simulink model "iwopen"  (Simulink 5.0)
settings: Solver=ode45  StartTime=0  StopTime=20  MaxStep=1e-3  RelTol=1e-3
undefined symbols (not defined in the file or in its folder): sat

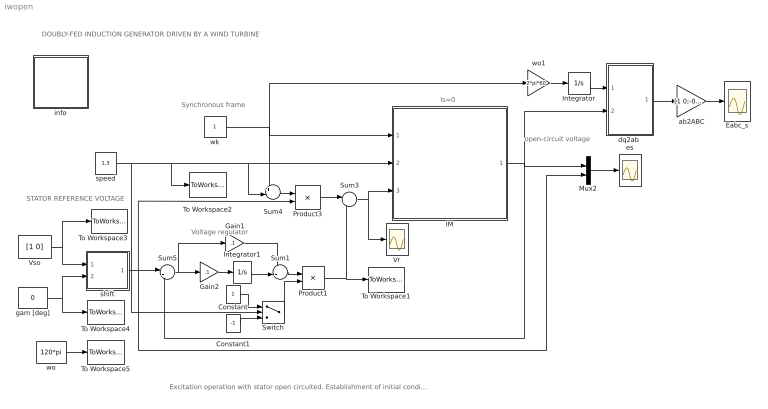
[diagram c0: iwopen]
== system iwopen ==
  note: STATOR REFERENCE VOLTAGE
  note: Synchronous frame
  note: DOUBLY-FED INDUCTION GENERATOR DRIVEN BY A WIND TURBINE
  note: Excitation operation with stator open circuited. Establishment of initial conditions.
  note: Is=0
  note: open-circuit voltage
  note: Voltage regulator
  Constant : Constant
  Constant1 : Constant  Value=-1
  Eabc_s : Scope
  Gain1 : Gain  Gain=.1
  Gain2 : Gain  Gain=.1
  IM : Subsystem  mask{Rr=.02, Lm=5, Lrl=0.1, wo=2*pi*60}
      mask prompts: Rr "Rotor resistance [pu]"; Lm "Magnetizing inductance [pu]"; Lrl "Rotor leakage inductance [pu]"; wo "base frequency [rad/s]"
  Integrator : Integrator
  Integrator1 : Integrator  UpperSaturationLimit=sat  LowerSaturationLimit=-sat
  Mux2 : Mux  Inputs=2
  Product1 : Product
  Product3 : Product
  Sum1 : Sum  Inputs=++|
  Sum3 : Sum  Inputs=|+-
  Sum4 : Sum  Inputs=+-|
  Sum5 : Sum  Inputs=|+-
  Switch : Switch  Criteria=u2 > Threshold  Threshold=1
  To Workspace1 : ToWorkspace  VariableName=vro  SampleTime=-1  SaveFormat=Array
  To Workspace2 : ToWorkspace  VariableName=wmo  SampleTime=-1  SaveFormat=Array
  To Workspace3 : ToWorkspace  VariableName=vso  SampleTime=-1  SaveFormat=Array
  To Workspace4 : ToWorkspace  VariableName=gamo  SampleTime=-1  SaveFormat=Array
  To Workspace5 : ToWorkspace  VariableName=wo  SampleTime=-1  SaveFormat=Array
  Vr : Scope
  Vso : Constant  Value=[1 0]
  ab2ABC : Gain  Gain=[1 0;-0.5 sqrt(3)/2;-0.5 -sqrt(3)/2]  Multiplication=Matrix(K*u)
  "dq2ab " : Subsystem
  es : Scope
  gam [deg] : Constant  Value=0
  info : Subsystem
  shift : Subsystem
  speed : Constant  Value=1.3
  wk : Constant
  wo : Constant  Value=120*pi
  wo1 : Gain  Gain=2*pi*60
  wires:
  IM/1(es) -> Sum5/2, Mux2/1, "dq2ab "/2(dq)
  Sum5/1 -> Gain2/1, Gain1/1
  speed/1 -> To Workspace2/1, IM/2(wm), Sum4/2, Switch/2
  wk/1 -> IM/1(wk), wo1/1, Sum4/1
  Vso/1 -> shift/1(vso), To Workspace3/1
  gam [deg]/1 -> shift/2(gama), To Workspace4/1
  wo/1 -> To Workspace5/1
  Gain2/1 -> Integrator1/1
  shift/1(vs) -> Mux2/2, Sum5/1, Product3/2
  Mux2/1 -> es/1
  Integrator1/1 -> Sum1/2
  Gain1/1 -> Sum1/1
  Constant/1 -> Switch/1
  Constant1/1 -> Switch/3
  Sum1/1 -> Product1/1
  Switch/1 -> Product1/2
  "dq2ab "/1(ab) -> ab2ABC/1
  ab2ABC/1 -> Eabc_s/1
  wo1/1 -> Integrator/1
  Integrator/1 -> "dq2ab "/1(thetas)
  Sum4/1 -> Product3/1
  Product3/1 -> Sum3/1
  Product1/1 -> Sum3/2, To Workspace1/1
  Sum3/1 -> IM/3(vr), Vr/1

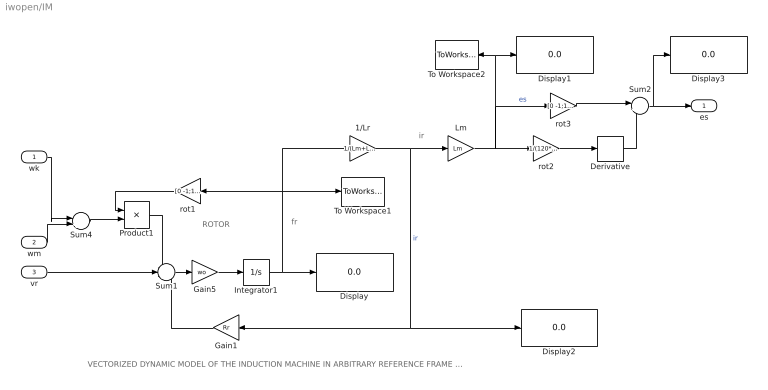
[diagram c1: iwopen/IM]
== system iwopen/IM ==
  note: ROTOR
  note: fr
  note: VECTORIZED DYNAMIC MODEL OF THE INDUCTION MACHINE IN ARBITRARY REFERENCE FRAME (stator open circuited --is=0)
  note: ir
  wk : Inport
  wm : Inport  Port=2
  vr : Inport  Port=3
  1/Lr : Gain  Gain=1/(Lm+Lrl)
  Derivative : Derivative
  Display{,1..3} (4 alike) : Display
  Gain1 : Gain  Orientation=left  Gain=Rr
  Gain5 : Gain  Gain=wo
  Integrator1 : Integrator  InitialCondition=[0 -1]
  Lm : Gain  Gain=Lm
  Product1 : Product
  Sum1 : Sum  Inputs=-+-
  Sum2 : Sum  Inputs=|++
  Sum4 : Sum  Inputs=|+-
  To Workspace1 : ToWorkspace  VariableName=fro  SampleTime=-1  SaveFormat=Array
  To Workspace2 : ToWorkspace  VariableName=fso  SampleTime=-1  SaveFormat=Array
  rot1 : Gain  Orientation=left  Gain=[0 -1;1 0]  Multiplication=Matrix(K*u)
  rot2 : Gain  Gain=1/(120*pi)  Multiplication=Matrix(K*u)
  rot3 : Gain  Gain=[0 -1;1 0]  Multiplication=Matrix(K*u)
  es : Outport
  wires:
  Gain1/1 -> Sum1/3
  Integrator1/1 -> rot1/1, To Workspace1/1, 1/Lr/1, Display/1
  Product1/1 -> Sum1/1
  rot1/1 -> Product1/1
  Sum4/1 -> Product1/2
  Sum1/1 -> Gain5/1
  Gain5/1 -> Integrator1/1
  wk/1 -> Sum4/1
  wm/1 -> Sum4/2
  vr/1 -> Sum1/2
  Lm/1 -> Display1/1, To Workspace2/1, rot3/1, rot2/1  "es"
  Sum2/1 -> es/1, Display3/1
  rot3/1 -> Sum2/1
  Derivative/1 -> Sum2/2
  rot2/1 -> Derivative/1
  1/Lr/1 -> Lm/1, Gain1/1, Display2/1  "ir"

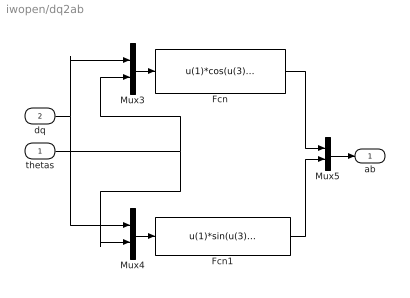
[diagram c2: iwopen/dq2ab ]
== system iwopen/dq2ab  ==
  thetas : Inport
  dq : Inport  Port=2
  Fcn : Fcn  Expr=u(1)*cos(u(3))-u(2)*sin(u(3))
  Fcn1 : Fcn  Expr=u(1)*sin(u(3))+u(2)*cos(u(3))
  Mux3 : Mux  Inputs=2
  Mux4 : Mux  Inputs=2
  Mux5 : Mux  Inputs=2
  ab : Outport
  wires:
  Mux3/1 -> Fcn/1
  Mux4/1 -> Fcn1/1
  dq/1 -> Mux3/1, Mux4/1
  thetas/1 -> Mux3/2, Mux4/2
  Fcn1/1 -> Mux5/2
  Fcn/1 -> Mux5/1
  Mux5/1 -> ab/1

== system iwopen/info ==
  note: The induction machine runs at a specified speed with the stator disconnected from the grid (is=0). The rotor is suddenly excited with slip-frequency voltages derived from voltage regulators so as to produce a commanded open-circuit stator terminal voltage. The induction machine is modeled in vectorized form in the synchronous frame . The specified operating conditions and the final values of the variables reached in a dc steady state are all saved in the workspace to serve as initial conditions in a subsequent simulation. This simulation deals with the connection of the stator to the grid.
  note: Doubly-Fed Induction Generator driven by a Wind Turbine Stator disconnected from grid

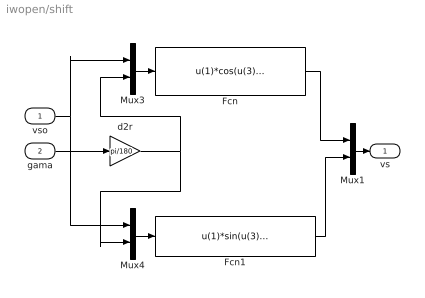
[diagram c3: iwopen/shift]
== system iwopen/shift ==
  vso : Inport
  gama : Inport  Port=2
  Fcn : Fcn  Expr=u(1)*cos(u(3))-u(2)*sin(u(3))
  Fcn1 : Fcn  Expr=u(1)*sin(u(3))+u(2)*cos(u(3))
  Mux1 : Mux  Inputs=2
  Mux3 : Mux  Inputs=2
  Mux4 : Mux  Inputs=2
  d2r : Gain  Gain=pi/180  Multiplication=Matrix(K*u)
  vs : Outport
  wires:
  Mux3/1 -> Fcn/1
  Mux4/1 -> Fcn1/1
  vso/1 -> Mux3/1, Mux4/1
  gama/1 -> d2r/1
  Fcn/1 -> Mux1/1
  Fcn1/1 -> Mux1/2
  d2r/1 -> Mux3/2, Mux4/2
  Mux1/1 -> vs/1
